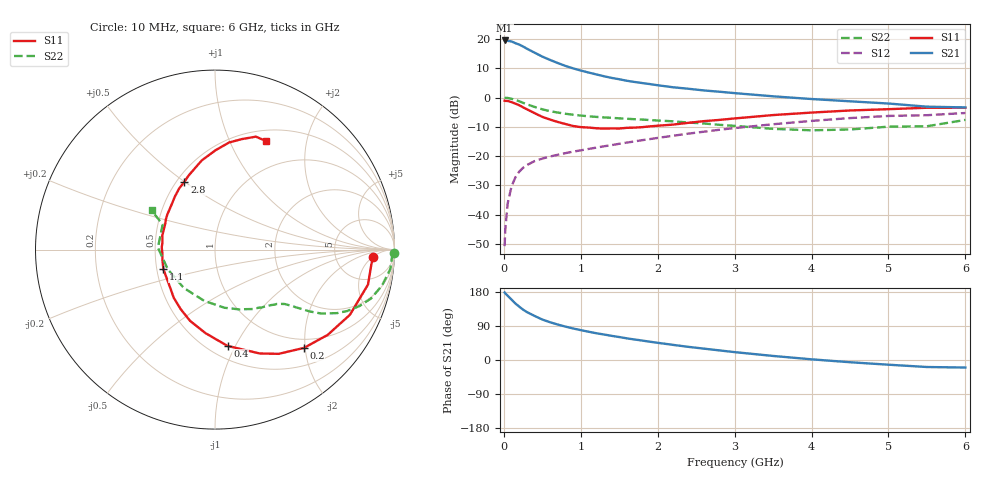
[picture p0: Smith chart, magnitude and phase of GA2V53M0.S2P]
! Infineon Technologies  Discrete & RF Semiconductors
! BF775
! Si NPN RF Bipolar Junction Transistor in SOT23
! VCE = 2.5 V  IC = 3 mA
! Common Emitter S-Parameters:  May  1996
# GHz  S  MA  R  50
!  f  S11  S21  S12  S22
! GHz  MAG  ANG  MAG  ANG  MAG  ANG  MAG  ANG
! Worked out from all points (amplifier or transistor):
!   36 points, 10 MHz to 6 GHz, reference 50 ohm
!   highest |S21| = 19.5 dB at 10 MHz (marker M1)
!   |S21| within 3 dB of that: start of sweep to 313.6 MHz
!   unconditionally stable (mu >= 1): 968.8 MHz to 3.903 GHz; 5.353 GHz to 5.787 GHz
!   at 250 MHz: K = 0.36, MSG = 20.7 dB, |S12| = -24.0 dB
!   at 1.4 GHz: K = 1.13, MAG = 9.3 dB, |S12| = -16.3 dB
!   at 6 GHz: K = 0.99, MSG = 1.0 dB, |S12| = -5.3 dB
!   S11 on the Smith chart (normalised r, x): 10 MHz: 14, -5; 200 MHz: 0.82, -1.97; 400 MHz: 0.61, -0.93; 1.1 GHz: 0.54, -0.13; 2.8 GHz: 0.55, +0.50; 6 GHz: 0.63, +1.37
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0.01  0.8821 -2.7  9.428 178.1  0.0029 85.7  0.995 -1.2
0.02  0.8752 -5.3  9.304 175.5  0.0059 86.2  0.9866 -2.5
0.05  0.8745 -12.9  9.281 169.5  0.0156 82.1  0.9828 -6.3
0.1  0.8348 -25.8  9.069 159.3  0.0304 75.9  0.9521 -12.1
0.15  0.7875 -37.1  8.47 149.1  0.0434 69.6  0.912 -17.3
0.2  0.7385 -47.9  8.025 140.8  0.0542 65.1  0.8636 -21.4
0.25  0.6804 -58.6  7.441 132.9  0.0631 60.6  0.8124 -24.9
0.3  0.6301 -66.7  6.818 126.5  0.0703 57.5  0.7663 -27.5
0.4  0.5412 -82.6  5.828 116.2  0.0822 53.0  0.6918 -31.0
0.5  0.468 -96.6  5.001 106.8  0.0907 50.6  0.6292 -33.2
0.6  0.4206 -109.3  4.391 99.7  0.0983 49.4  0.585 -34.4
0.7  0.383 -119.9  3.885 93.6  0.1053 48.8  0.5542 -35.5
0.9  0.3267 -140.1  3.146 83.2  0.1192 48.4  0.5091 -37.2
1.1  0.3074 -159.2  2.675 74.7  0.1324 49.3  0.4787 -39.2
1.3  0.294 -175.2  2.312 67.3  0.147 49.7  0.4576 -41.5
1.6  0.3039 165.0  1.932 57.1  0.1702 49.8  0.4338 -45.9
2.2  0.345 135.3  1.497 39.9  0.2226 48.6  0.3927 -57.5
2.8  0.4148 114.3  1.257 25.4  0.2816 44.6  0.3421 -73.8
3.5  0.502 98.5  1.049 10.7  0.3499 37.4  0.2917 -101.9
4.5  0.6013 82.6  0.862 -5.9  0.446 24.7  0.2849 -157.1
5.5  0.6692 70.1  0.698 -18.5  0.4993 9.5  0.3235 154.4
6  0.6683 65.0  0.678 -19.9  0.5444 5.4  0.4148 148.3
